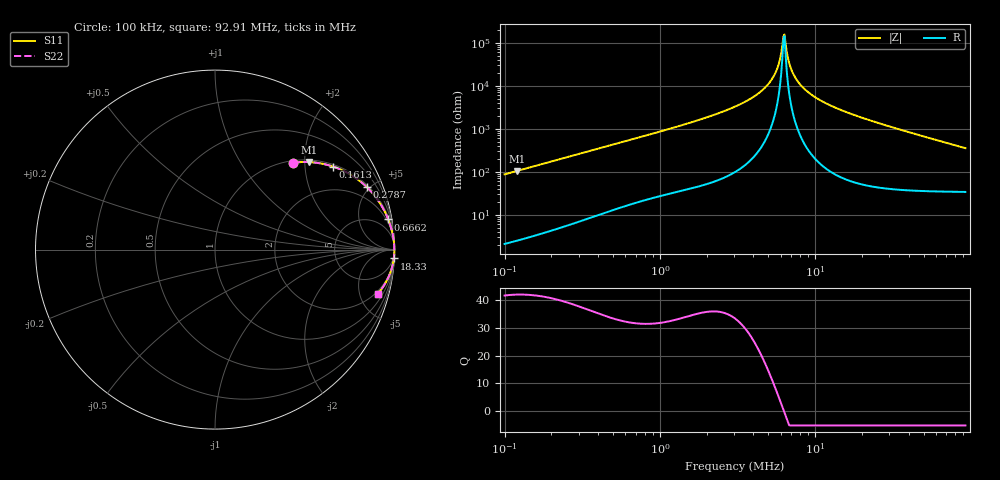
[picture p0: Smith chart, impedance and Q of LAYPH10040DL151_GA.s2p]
! LAYPH10040DL151_GA  S-PARAMETER MODEL  ( General Type )
! Model Generated by TAIYO YUDEN Corporation (http://www.ty-top.com)
! Version 1.0
! TAIYO YUDEN Control No. 180920NI43SB-FBB
! Copyright(c) 2018 TAIYO YUDEN CO.,LTD. All Rights Reserved.
! Product Description (link to TY-COMPAS)
! https://ds.yuden.co.jp/TYCOMPAS/or/detail?pn=LAYPH10040DL151MGA&u=M
! Products Name : Inductors
! Characteristics :
!  Inductance : 150 uH , SRF(min) : -Hz , DC Resistance(max) : 0.474 Ohm
!  Rated Current : Saturation :0.94 A , Temp Rise : 0.44 A (25 degC)
!  Case Size : 10.1 x 10.0 / 0.398 x 0.394 [mm/inch] , Thickness : 4 / 0.157 [mm/inch]
!  (Conditions: Temperature = 25 degC , DC Bias Current/Voltage = 0A / 0V)
! External Node Assignments :
!  1  o---GGG---o  2
! GND o---------o GND
! Frequency Range : 0.1MHz  -  92.907885MHz  [ 402 STEP ]
# MHz S RI R 50
! Freq[MHz].  S11 Real  S11 Imag  S21 Real  S21 Imag  S12 Real  S12 Imag  S22 Real  S22 Imag
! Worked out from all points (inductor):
!   401 points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, 100 kHz to 92.91 MHz, reference 50 ohm
!   read as one part in series: L = 138 uH near 103.5 kHz
!   highest Q = 41.8 at 120.7 kHz (marker M1), where L = 139 uH
!   self-resonance near 6.247 MHz
!   S11 on the Smith chart (normalised r, x): 100 kHz: 1.04, +1.75; 161.3 kHz: 1.07, +2.80; 278.7 kHz: 1.13, +4.81; 666.2 kHz: 1, +11; 18.33 MHz: 2, -40; 92.91 MHz: 1.68, -7.07
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0.1  0.434 0.4837  0.566 -0.4837  0.566 -0.4837  0.434 0.4837
0.120676  0.5245 0.4876  0.4755 -0.4876  0.4755 -0.4876  0.5245 0.4876
0.161348  0.659 0.4621  0.341 -0.4621  0.341 -0.4621  0.659 0.4621
0.278746  0.8464 0.3477  0.1536 -0.3477  0.1536 -0.3477  0.8464 0.3477
0.314158  0.8736 0.3191  0.1264 -0.3191  0.1264 -0.3191  0.8736 0.3191
0.666246  0.9652 0.168  0.0348 -0.168  0.0348 -0.168  0.9652 0.168
0.986956  0.9828 0.1153  0.0172 -0.1153  0.0172 -0.1153  0.9828 0.1153
3.100605  0.9982 0.0296  0.00178 -0.0296  0.00178 -0.0296  0.9982 0.0296
4.145612  0.999 0.0166  0.000973 -0.0166  0.000973 -0.0166  0.999 0.0166
5.088974  0.9993 0.00835  0.000689 -0.00835  0.000689 -0.00835  0.9993 0.00835
5.638337  0.9994 0.00435  0.000617 -0.00435  0.000617 -0.00435  0.9994 0.00435
5.834334  0.9994 0.00303  0.000603 -0.00303  0.000603 -0.00303  0.9994 0.00303
6.141178  0.9994 0.00106  0.00059 -0.00106  0.00059 -0.00106  0.9994 0.00106
6.354654  0.9994 -0.000255  0.000587 0.000255  0.000587 0.000255  0.9994 -0.000255
6.46416  0.9994 -0.000913  0.000587 0.000913  0.000587 0.000913  0.9994 -0.000913
6.921378  0.9994 -0.00355  0.0006 0.00355  0.0006 0.00355  0.9994 -0.00355
7.285393  0.9994 -0.00553  0.000622 0.00553  0.000622 0.00553  0.9994 -0.00553
8.21096  0.9993 -0.0102  0.000715 0.0102  0.000715 0.0102  0.9993 -0.0102
9.575801  0.9991 -0.0165  0.000932 0.0165  0.000932 0.0165  0.9991 -0.0165
18.32906  0.9962 -0.0491  0.00377 0.0491  0.00377 0.0491  0.9962 -0.0491
30.08319  0.9893 -0.0866  0.0107 0.0866  0.0107 0.0866  0.9893 -0.0866
92.90788  0.9062 -0.2474  0.0938 0.2474  0.0938 0.2474  0.9062 -0.2474
